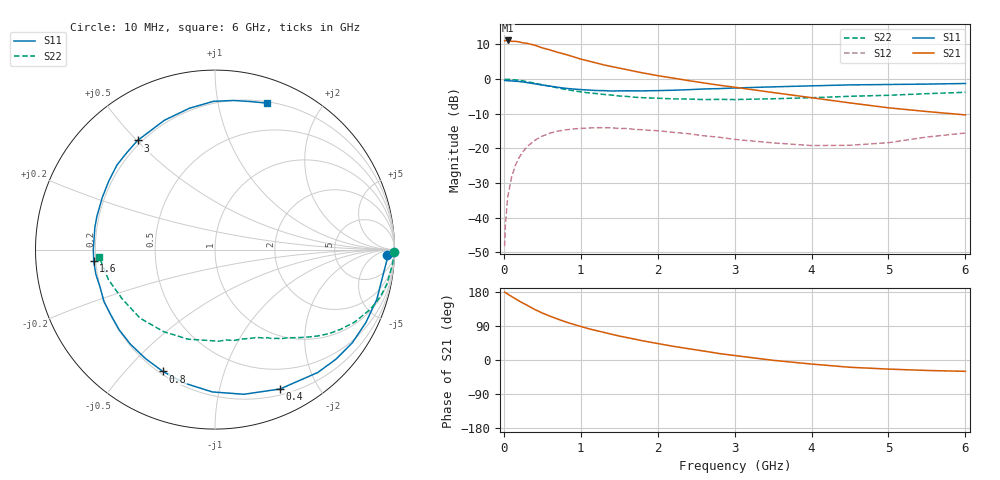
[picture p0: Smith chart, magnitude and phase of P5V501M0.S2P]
! SIEMENS Small Signal Semiconductors
! BFP183
! Si NPN RF Bipolar Junction Transistor in SOT143
! VCE = 0.5 V  IC = 1 mA
! Common Emitter S-Parameters:  March  1996
# GHz  S  MA  R  50
!  f  S11  S21  S12  S22
! GHz  MAG  ANG  MAG  ANG  MAG  ANG  MAG  ANG
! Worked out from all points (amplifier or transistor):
!   36 points, 10 MHz to 6 GHz, reference 50 ohm
!   highest |S21| = 11.2 dB at 50 MHz (marker M1)
!   |S21| within 3 dB of that: start of sweep to 639 MHz
!   unconditionally stable (mu >= 1): 2.256 GHz to end of sweep
!   at 250 MHz: K = 0.12, MSG = 15.7 dB, |S12| = -20.9 dB
!   at 1.4 GHz: K = 0.61, MSG = 8.8 dB, |S12| = -14.0 dB
!   at 6 GHz: K = 1.41, MAG = -1.2 dB, |S12| = -15.5 dB
!   S11 on the Smith chart (normalised r, x): 10 MHz: 31, -21; 400 MHz: 0.26, -1.54; 800 MHz: 0.21, -0.64; 1.6 GHz: 0.19, -0.05; 3 GHz: 0.18, +0.50; 6 GHz: 0.21, +1.39
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0.01  0.9568 -1.7  3.554 179.2  0.0039 85.5  0.9989 -0.8
0.02  0.9593 -3.6  3.605 178.2  0.0078 89.2  0.9898 -1.5
0.05  0.9469 -8.6  3.614 173.9  0.0199 85.3  0.9945 -3.8
0.1  0.9433 -17.1  3.511 167.8  0.0383 79.7  0.9843 -7.6
0.15  0.9336 -25.8  3.512 161.6  0.057 73.9  0.9758 -11.5
0.2  0.9246 -34.2  3.445 155.5  0.0745 69.0  0.9615 -15.0
0.3  0.8926 -50.1  3.287 144.7  0.1056 59.6  0.9226 -21.5
0.4  0.857 -65.0  3.089 133.5  0.1308 50.8  0.877 -27.4
0.5  0.822 -78.7  2.825 124.0  0.1507 43.0  0.8298 -32.3
0.6  0.7931 -91.1  2.64 115.7  0.1667 36.1  0.789 -36.4
0.7  0.7634 -102.8  2.436 108.0  0.1776 30.2  0.7483 -40.0
0.8  0.7383 -113.2  2.278 100.8  0.1852 24.9  0.713 -43.1
0.9  0.7202 -122.5  2.109 94.5  0.1913 20.1  0.6812 -46.0
1.1  0.6963 -140.1  1.828 82.7  0.1974 11.9  0.6344 -50.8
1.4  0.6738 -161.7  1.519 68.0  0.1986 1.6  0.5891 -57.4
1.6  0.6789 -174.5  1.371 59.2  0.1939 -3.2  0.564 -60.9
2.2  0.6917 155.3  1.036 36.2  0.1712 -14.0  0.5196 -73.6
3  0.7455 125.3  0.765 11.8  0.1354 -19.6  0.5076 -93.4
3.5  0.7739 111.3  0.641 -0.8  0.1203 -16.1  0.5213 -106.8
4.5  0.8261 90.6  0.454 -19.2  0.1112 -0.5  0.5659 -137.6
5.5  0.8482 76.5  0.341 -27.6  0.1463 10.3  0.6173 -164.4
6  0.8656 70.5  0.305 -29.9  0.1671 8.9  0.6464 -176.4
